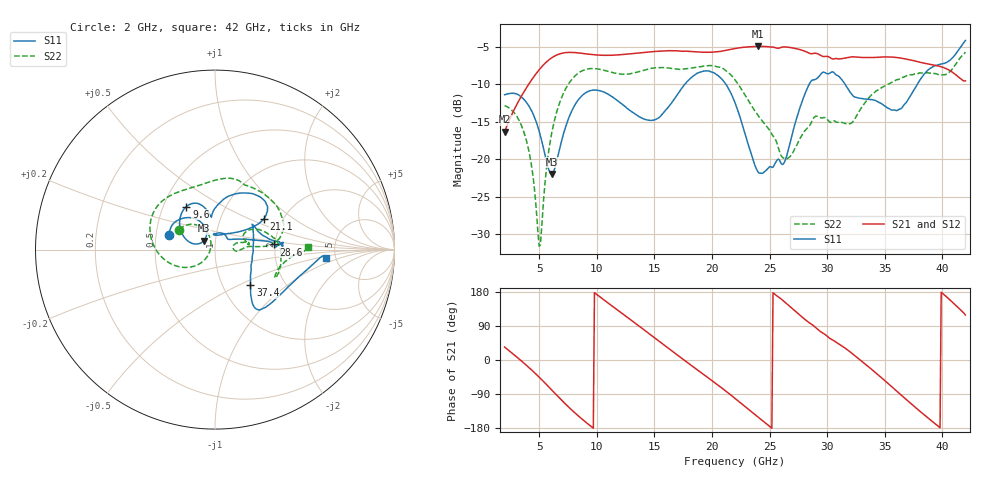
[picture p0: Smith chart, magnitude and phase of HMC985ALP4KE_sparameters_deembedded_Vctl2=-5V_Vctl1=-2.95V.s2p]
!s2p File: Measurements: S11, S21, S12, S22
# GHz S dB R 50.0
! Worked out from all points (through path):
!   401 points, 2 GHz to 42 GHz, reference 50 ohm
!   highest |S21| = -4.96 dB at 24 GHz (marker M1); lowest = -16.3 dB at 2 GHz (marker M2)
!   lowest |S11| = -22.0 dB at 6.1 GHz (marker M3), VSWR 1.17, Z = 43.9 + j4.4 ohm
!   |S11| at or under -10 dB: start of sweep to 17.66 GHz; 21.2 GHz to 28.45 GHz (7.241 GHz wide, 29.2 % of centre); 31.55 GHz to 37.83 GHz (6.286 GHz wide, 18.1 % of centre)
!   |S22| runs from -31.6 to -5.7 dB; largest |S21 - S12| = 0.0006
!   S11 on the Smith chart (normalised r, x): 2 GHz: 0.59, +0.11; 9.6 GHz: 0.65, +0.34; 21.1 GHz: 1.61, +0.62; 28.6 GHz: 1.98, +0.13; 37.4 GHz: 1.35, -0.57; 42 GHz: 4.13, -0.65
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2  -11.41 162.0  -16.34 34.2  -16.35 34.2  -12.85 150.8
3.9  -12.44 131.8  -10.47 -14.1  -10.48 -14.1  -17.54 118.5
5  -16.26 115.1  -8.08 -45.3  -8.09 -45.3  -31.59 156.7
6.1  -21.98 141.4  -6.48 -79.4  -6.48 -79.4  -16.43 -141.9
7.2  -16.15 162.8  -5.82 -113.6  -5.82 -113.6  -10.91 -168.3
8.7  -11.56 137.2  -5.89 -155.4  -5.89 -155.4  -8.25 159.2
9.6  -10.81 123.7  -6.06 -177.6  -6.06 -177.6  -7.91 144.4
12.8  -13.41 100.4  -5.97 109.3  -5.98 109.3  -8.65 102.1
15.4  -14.46 95.7  -5.62 49.7  -5.62 49.7  -7.79 75.1
18  -9.42 67.9  -5.62 -9.6  -5.62 -9.6  -7.90 59.1
21.1  -9.79 32.3  -5.52 -79.5  -5.52 -79.5  -8.07 16.4
22  -12.46 31.1  -5.25 -101.3  -5.26 -101.3  -9.42 6.9
24  -21.70 77.2  -4.96 -150.2  -4.96 -150.2  -14.16 5.3
26.4  -19.99 34.4  -5.04 150.4  -5.05 150.4  -19.95 6.2
28.6  -9.61 5.0  -5.95 95.2  -5.95 95.3  -15.20 14.4
28.7  -9.46 3.6  -5.93 93.2  -5.94 93.2  -14.85 14.3
30.5  -8.36 5.5  -6.65 52.3  -6.66 52.3  -14.92 14.7
32.4  -11.72 23.7  -6.37 11.3  -6.37 11.3  -14.64 28.8
35.4  -13.28 9.1  -6.38 -64.9  -6.38 -64.9  -9.95 14.4
37.4  -11.11 -44.7  -6.84 -118.4  -6.84 -118.3  -8.75 -2.2
39.7  -7.38 -48.7  -7.59 -176.2  -7.60 -176.2  -8.72 -24.9
42  -4.18 -4.5  -9.56 118.6  -9.57 118.6  -5.73 1.8
